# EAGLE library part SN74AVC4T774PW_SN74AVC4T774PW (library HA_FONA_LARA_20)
Check prices
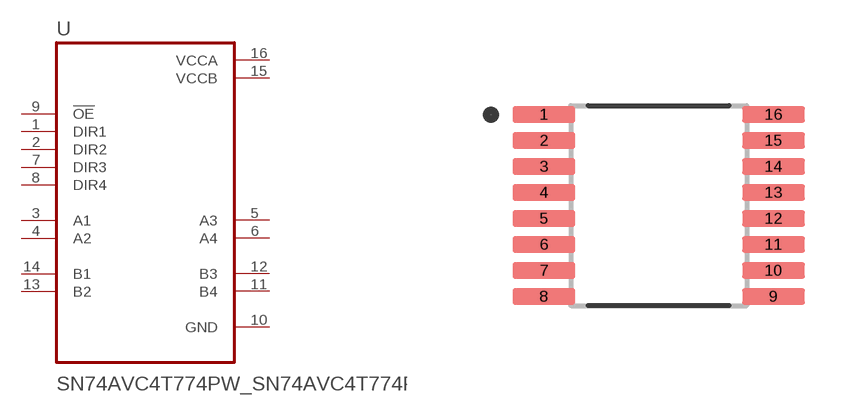
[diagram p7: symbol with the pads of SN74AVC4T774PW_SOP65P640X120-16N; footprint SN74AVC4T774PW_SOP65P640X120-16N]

Designator prefix U

## SN74AVC4T774PW_SN74AVC4T774PW (AVAILABILITY: Good; DESCRIPTION: 4-bit dual-supply bus transceiver with configurable voltage-level shifting and 3-state outputs 16-TSSOP -40 to 85; MF: Texas Instruments; MP: SN74AVC4T774PW; PACKAGE: TSSOP-16 Texas Instruments; PRICE: None; PURCHASE-URL: https://pricing.snapeda.com/search/part/SN74AVC4T774PW/?ref=eda)  [SN74AVC4T774PW_SOP65P640X120-16N]
1  DIR1  in
2  DIR2  in
3  A1
4  A2
5  A3
6  A4
7  DIR3  in
8  DIR4  in
9  !OE  in
10  GND  pwr
11  B4
12  B3
13  B2
14  B1
15  VCCB  pwr
16  VCCA  pwr

## Footprint SN74AVC4T774PW_SOP65P640X120-16N (pad centres in mm)
smd 1.57 x 0.41: 1 -2.87,2.275; 2 -2.87,1.625; 3 -2.87,0.975; 4 -2.87,0.325; 5 -2.87,-0.325; 6 -2.87,-0.975; 7 -2.87,-1.625; 8 -2.87,-2.275; 9 2.87,-2.275; 10 2.87,-1.625; 11 2.87,-0.975; 12 2.87,-0.325; 13 2.87,0.325; 14 2.87,0.975; 15 2.87,1.625; 16 2.87,2.275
